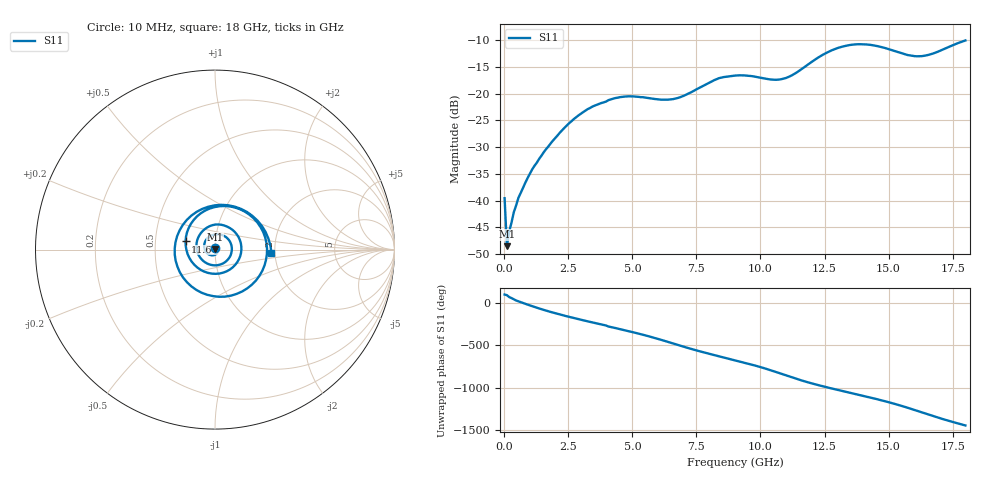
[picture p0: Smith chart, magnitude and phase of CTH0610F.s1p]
!Agilent Technologies,N5224A,MY51441447,A.10.00.00
!Agilent N5224A: A.10.00.00
!Date: Thursday, January 07, 2016 10:57:20
!Correction: S11(Full 1 Port(1))
!S1P File: Measurement: S11:
# Hz S  RI  R 50
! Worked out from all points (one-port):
!   201 points, 10 MHz to 18 GHz, reference 50 ohm
!   lowest |S11| = -48.5 dB at 99.95 MHz (marker M1), VSWR 1.01, Z = 50 + j0.375 ohm
!   |S11| at or under -10 dB: start of sweep to end of sweep
!   S11 on the Smith chart (normalised r, x): 10 MHz: 1.00, +0.02; 11.61 GHz: 0.72, +0.07; 18 GHz: 1.92, -0.07
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1e7  -0.000636 0.0105
9.995e7  0.000277 0.00374
3.698e8  0.0062 0.00476
8.1955e8  0.0142 -0.00387
2.25875e9  -0.0386 -0.0244
3.2482e9  -0.0542 0.0468
4.5075e9  0.0619 0.0691
5.49695e9  0.0833 -0.039
6.75625e9  -0.066 -0.0627
7.7457e9  -0.0874 0.0791
8.37535e9  0.00258 0.1396
9.005e9  0.11 0.0986
9.63465e9  0.1452 -0.0178
1.035425e10  0.0449 -0.1286
1.125375e10  -0.1421 -0.0474
1.161355e10  -0.1642 0.0455
1.20633e10  -0.119 0.1648
1.2603e10  0.0251 0.2416
1.305275e10  0.1675 0.2109
1.35025e10  0.2683 0.0982
1.413215e10  0.2634 -0.1185
1.47618e10  0.0888 -0.2566
1.521155e10  -0.075 -0.2401
1.575125e10  -0.2094 -0.0945
1.629095e10  -0.1973 0.1072
1.69206e10  -0.000296 0.2468
1.737035e10  0.1781 0.2096
1.8e10  0.3143 -0.0162
